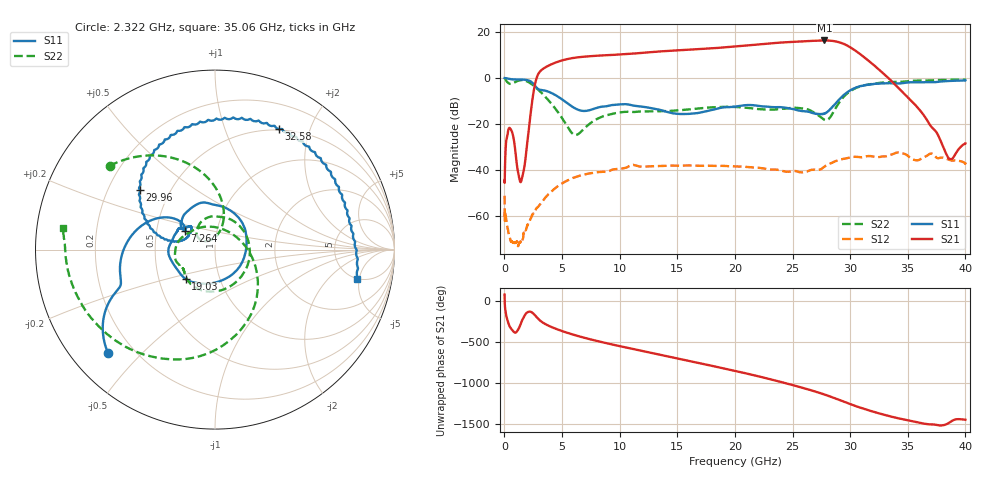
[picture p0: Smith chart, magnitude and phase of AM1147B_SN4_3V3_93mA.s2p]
!Agilent Technologies,E8363B,US42420178,A.07.50.48
!Agilent E8363B: A.07.50.48
!Date: Thursday, November 17, 2022 08:48:29
!Correction: S11(Full 2 Port(1,2))
!S21(Full 2 Port(1,2))
!S12(Full 2 Port(1,2))
!S22(Full 2 Port(1,2))
!S2P File: Measurements: S11, S21, S12, S22:
# Hz S  dB  R 50
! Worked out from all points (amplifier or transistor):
!   6401 points, 10 MHz to 40 GHz, reference 50 ohm
!   highest |S21| = 16.3 dB at 27.77 GHz (marker M1)
!   |S21| within 3 dB of that: 19.08 GHz to 30.02 GHz (10.94 GHz wide, 44.5 % of centre)
!   unconditionally stable (mu >= 1): 18.4 MHz to 27.83 MHz; 52.21 MHz to end of sweep
!   at 6.671 GHz: K = 21.28, MAG = 9.4 dB, |S12| = -42.1 dB
!   at 20 GHz: K = 7.64, MAG = 14.2 dB, |S12| = -38.3 dB
!   at 40 GHz: K = 31.68, MAG = -13.7 dB, |S12| = -36.9 dB
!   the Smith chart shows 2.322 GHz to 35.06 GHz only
!   S11 on the Smith chart (normalised r, x): 2.322 GHz: 0.11, -0.40; 7.264 GHz: 0.70, +0.15; 19.03 GHz: 0.69, -0.24; 29.96 GHz: 0.34, +0.31; 32.58 GHz: 0.49, +1.55; 35.06 GHz: 4.75, -4.59
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1e7  -0.00 -0.3  -44.38 74.7  -51.01 52.6  0.02 -2.6
2.321922e9  -1.62 -135.8  -13.17 -137.3  -60.38 -125.5  -2.50 141.5
3.784056e9  -5.84 -179.6  5.29 59.2  -50.52 149.5  -9.44 88.6
6.677083e9  -14.15 146.2  9.17 -80.1  -42.13 31.5  -23.08 138.5
7.264436e9  -14.06 148.6  9.43 -101.9  -41.44 11.8  -20.30 145.9
1.012622e10  -11.36 113.9  10.30 165.0  -39.24 -67.9  -14.81 105.4
1.334417e10  -13.61 40.4  11.51 69.2  -38.15 -163.2  -14.38 26.4
1.612472e10  -15.48 -53.9  12.37 -13.9  -37.88 115.0  -13.51 -48.2
1.903024e10  -12.70 -134.9  13.30 -101.0  -38.08 31.2  -12.46 -106.8
2.0005e10  -12.37 -156.1  13.69 -131.1  -38.30 2.6  -12.53 -121.7
2.206074e10  -12.04 171.6  14.65 162.3  -38.90 -54.6  -13.45 -143.4
2.403524e10  -12.62 150.0  15.44 92.9  -40.14 -115.3  -13.35 -154.7
2.523494e10  -13.70 143.2  15.77 48.3  -40.26 -153.9  -12.87 -169.1
2.667208e10  -14.98 137.6  16.13 -8.9  -39.76 152.6  -14.37 157.0
2.777181e10  -15.43 156.7  16.32 -57.6  -38.35 108.3  -18.11 86.2
2.871532e10  -11.07 168.2  15.93 -105.3  -36.02 57.2  -13.24 -14.2
2.995876e10  -5.45 141.7  13.50 -172.1  -34.43 -6.8  -5.84 -80.3
3.103974e10  -3.30 110.8  9.73 135.3  -34.34 -53.0  -3.39 -116.6
3.257686e10  -2.39 62.2  3.35 70.8  -34.20 -105.6  -2.08 -150.7
3.333917e10  -2.22 40.3  -0.08 42.4  -33.58 -126.8  -1.78 -163.9
3.506373e10  -1.88 -12.2  -8.62 -12.4  -33.96 163.9  -1.33 171.7
4e10  -1.00 -140.7  -28.32 -4.4  -36.93 29.6  -0.81 110.7
